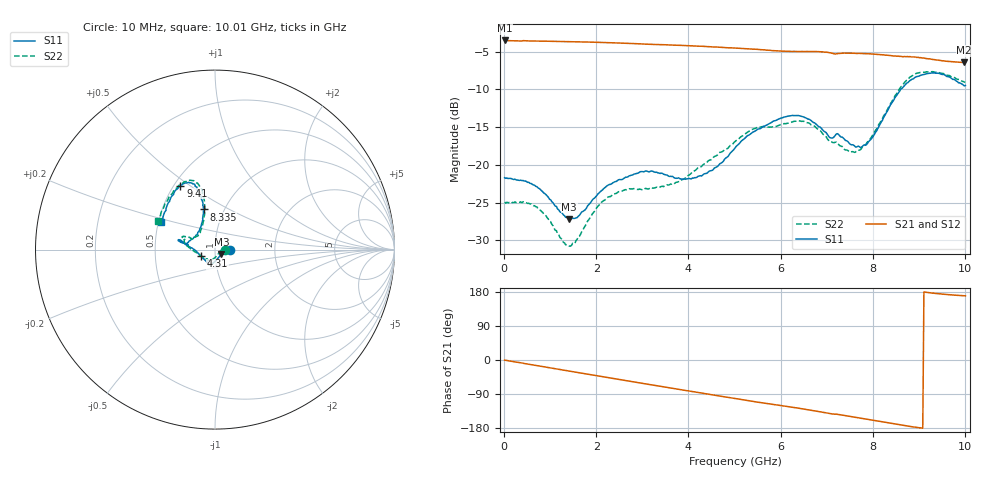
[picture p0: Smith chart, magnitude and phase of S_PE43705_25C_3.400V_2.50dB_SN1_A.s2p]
! Device ID: PE43705
! Serial: 1
! Insertion: A
! Impedance: 50 ohm
! Temp: 25C
! VDD: 3.400V
! Attenuation Step: 2.50dB
#  Hz  S  RI  R  50
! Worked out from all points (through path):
!   401 points, 10 MHz to 10.01 GHz, reference 50 ohm
!   highest |S21| = -3.52 dB at 10 MHz (marker M1); lowest = -6.4 dB at 9.985 GHz (marker M2)
!   group delay of S21, straight-line fit = 54.2 ps
!   lowest |S11| = -27.2 dB at 1.41 GHz (marker M3), VSWR 1.09, Z = 53.7 - j2.67 ohm
!   |S11| at or under -10 dB: start of sweep to 8.605 GHz
!   |S22| runs from -30.8 to -7.6 dB; largest |S21 - S12| = 0.0062
!   S11 on the Smith chart (normalised r, x): 10 MHz: 1.18, -0.00; 4.31 GHz: 0.85, -0.06; 8.335 GHz: 0.80, +0.38; 9.41 GHz: 0.54, +0.46; 10.01 GHz: 0.52, +0.18
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1e7  0.0823 -0.000546  0.667 -0.00316  0.6675 -0.00303  0.0567 -0.000155
6.6e8  0.0728 0.00954  0.6422 -0.1576  0.642 -0.1573  0.0519 0.0137
1.41e9  0.0362 -0.0249  0.5717 -0.3203  0.5721 -0.3201  0.0235 -0.0171
1.685e9  0.0202 -0.0446  0.5352 -0.3735  0.5352 -0.3735  0.00902 -0.0351
2.285e9  -0.00865 -0.0738  0.4379 -0.4729  0.4383 -0.4727  -0.0192 -0.0586
2.96e9  -0.0311 -0.0847  0.3075 -0.5533  0.3079 -0.553  -0.0401 -0.0562
3.36e9  -0.0376 -0.08  0.2265 -0.5839  0.2271 -0.5834  -0.0463 -0.0538
4.31e9  -0.0769 -0.0377  0.0236 -0.6097  0.024 -0.6097  -0.0976 -0.021
5.01e9  -0.1291 0.00928  -0.1193 -0.5814  -0.1188 -0.5818  -0.1425 0.0102
5.435e9  -0.1642 0.029  -0.1985 -0.5491  -0.1981 -0.55  -0.1692 0.0393
6.035e9  -0.1979 0.0544  -0.2894 -0.4873  -0.2875 -0.4879  -0.1765 0.0617
6.685e9  -0.1895 0.0404  -0.3849 -0.411  -0.3852 -0.4107  -0.1676 0.0733
7.085e9  -0.1488 0.0268  -0.4327 -0.3433  -0.4331 -0.3435  -0.1308 0.0595
7.26e9  -0.1544 0.0361  -0.4417 -0.3227  -0.4404 -0.3236  -0.1184 0.0673
7.61e9  -0.1134 0.0694  -0.4794 -0.2664  -0.4785 -0.267  -0.088 0.0831
7.91e9  -0.0846 0.115  -0.5004 -0.2123  -0.5007 -0.215  -0.0745 0.1245
8.335e9  -0.0636 0.2236  -0.5148 -0.1317  -0.5138 -0.1347  -0.056 0.2317
8.36e9  -0.0647 0.2333  -0.5157 -0.1268  -0.515 -0.1291  -0.0575 0.2408
8.86e9  -0.1111 0.3535  -0.5179 -0.0337  -0.5149 -0.0375  -0.1077 0.3745
9.41e9  -0.1927 0.356  -0.4926 0.0427  -0.4915 0.0421  -0.1963 0.3627
9.985e9  -0.2912 0.1629  -0.4689 0.0865  -0.4702 0.0865  -0.3092 0.1711
1.001e10  -0.2988 0.1527  -0.47 0.0882  -0.4724 0.0878  -0.3165 0.1589
